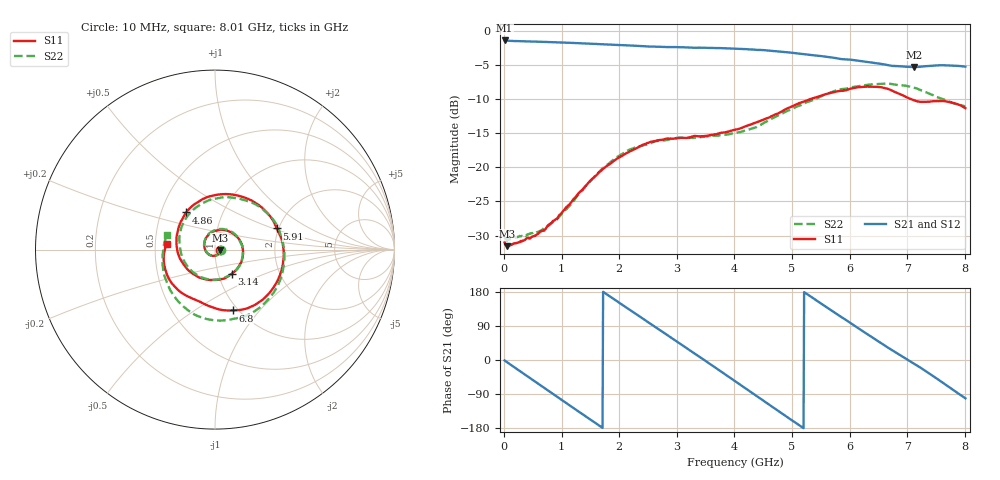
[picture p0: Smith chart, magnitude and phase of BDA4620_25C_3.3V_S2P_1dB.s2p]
!Agilent Technologies,E5071B,MY42404982,A.09.10
!Date: Wed May 06 08:56:10 2026
!Data & Calibration Information:
!Freq	S11:SOLT2(ON)	S21:SOLT2(ON)	S12:SOLT2(ON)	S22:SOLT2(ON)
# Hz S RI R 50
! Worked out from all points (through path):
!   801 points, 10 MHz to 8.01 GHz, reference 50 ohm
!   highest |S21| = -1.45 dB at 10 MHz (marker M1); lowest = -5.3 dB at 7.12 GHz (marker M2)
!   group delay of S21, straight-line fit = 285 ps
!   lowest |S11| = -31.6 dB at 60 MHz (marker M3), VSWR 1.05, Z = 52.7 - j0.41 ohm
!   |S11| at or under -10 dB: start of sweep to 5.33 GHz; 7.057 GHz to end of sweep
!   |S22| runs from -30.7 to -7.8 dB; largest |S21 - S12| = 0.0037
!   S11 on the Smith chart (normalised r, x): 10 MHz: 1.06, -0.00; 3.14 GHz: 1.16, -0.32; 4.86 GHz: 0.67, +0.30; 5.91 GHz: 1.96, +0.53; 6.8 GHz: 0.94, -0.73; 8.01 GHz: 0.58, +0.04
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1e7  0.028 -0.00196  0.8461 -0.0179  0.8469 -0.0178  0.0307 -0.00192
6e7  0.0261 -0.00389  0.8366 -0.0968  0.8387 -0.0981  0.0291 -0.00344
3.7e8  0.0204 -0.0214  0.6457 -0.5277  0.646 -0.5288  0.0232 -0.0215
7.3e8  -0.00897 -0.0347  0.1853 -0.804  0.1852 -0.805  -0.00595 -0.0361
1.03e9  -0.0444 -0.0182  -0.257 -0.775  -0.2581 -0.7757  -0.0423 -0.0206
1.35e9  -0.0604 0.0315  -0.6333 -0.4994  -0.6335 -0.5  -0.0606 0.0288
1.93e9  0.0253 0.1102  -0.7301 0.2907  -0.7311 0.2916  0.0216 0.114
2.32e9  0.1162 0.0767  -0.3632 0.6815  -0.3644 0.6822  0.1153 0.0816
2.68e9  0.1568 -0.0165  0.1124 0.7526  0.1135 0.7535  0.1555 -0.00457
3.14e9  0.0951 -0.1334  0.622 0.4257  0.6234 0.4248  0.108 -0.1239
3.57e9  -0.0248 -0.1687  0.7353 -0.1274  0.7358 -0.1289  -0.0123 -0.1688
4.01e9  -0.1514 -0.1113  0.4151 -0.6093  0.4148 -0.6103  -0.143 -0.1061
4.43e9  -0.2147 0.03  -0.1199 -0.711  -0.1212 -0.7118  -0.1976 0.0365
4.86e9  -0.1602 0.2067  -0.5697 -0.4028  -0.5705 -0.4026  -0.1271 0.2163
5.35e9  0.0773 0.3091  -0.637 0.173  -0.6375 0.1738  0.1137 0.2867
5.91e9  0.3445 0.1178  -0.1928 0.585  -0.193 0.586  0.3654 0.0806
6.26e9  0.3714 -0.1128  0.1752 0.5663  0.1769 0.5668  0.3726 -0.1394
6.68e9  0.1751 -0.3286  0.4752 0.2891  0.4768 0.2892  0.1964 -0.3578
6.8e9  0.0988 -0.3391  0.5157 0.1904  0.5177 0.19  0.1176 -0.3832
7.12e9  -0.0598 -0.303  0.5324 -0.0938  0.5336 -0.0952  -0.0982 -0.3692
7.62e9  -0.2462 -0.1803  0.2766 -0.4829  0.2768 -0.4845  -0.2832 -0.1379
8.01e9  -0.2688 0.0311  -0.1049 -0.5342  -0.106 -0.5356  -0.2657 0.0832
